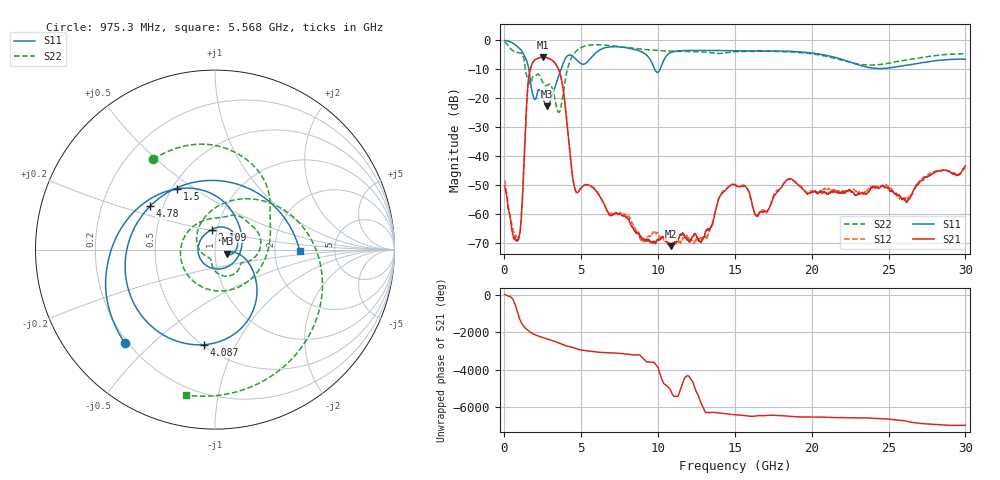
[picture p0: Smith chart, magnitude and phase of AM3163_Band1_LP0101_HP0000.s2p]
!Agilent Technologies,E8364B,MY43040894,A.07.50.67
!Agilent E8364B: A.07.50.67
!Date: Thursday, August 20, 2020 11:26:09
!Correction: S11(Full 2 Port(1,2))
!S21(Full 2 Port(1,2))
!S12(Full 2 Port(1,2))
!S22(Full 2 Port(1,2))
!S2P File: Measurements: S11, S21, S12, S22:
# Hz S  dB  R 50
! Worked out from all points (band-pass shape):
!   3201 points, 10 MHz to 30 GHz, reference 50 ohm
!   highest |S21| = -5.82 dB at 2.512 GHz (marker M1); lowest = -71.3 dB at 10.86 GHz (marker M2)
!   |S21| within 3 dB of the highest: 1.752 GHz to 3.411 GHz (1.659 GHz wide, 64.3 % of centre)
!   lowest |S11| = -22.8 dB at 2.775 GHz (marker M3), VSWR 1.16, Z = 57.4 - j2.53 ohm
!   |S11| at or under -10 dB: 1.588 GHz to 3.688 GHz (2.099 GHz wide, 79.6 % of centre); 9.776 GHz to 10.13 GHz (355.8 MHz wide, 3.57 % of centre)
!   |S22| runs from -24.9 to -0.6 dB; largest |S21 - S12| = 0.0029
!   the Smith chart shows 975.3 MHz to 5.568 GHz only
!   S11 on the Smith chart (normalised r, x): 975.3 MHz: 0.19, -0.41; 1.5 GHz: 0.53, +0.43; 2.109 GHz: 0.94, +0.21; 4.087 GHz: 0.51, -0.75; 4.78 GHz: 0.42, +0.25; 5.568 GHz: 2.79, -0.06
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1e7  -0.07 -8.8  -50.49 19.2  -48.45 10.2  -0.56 -25.3
5.067094e8  -0.89 -67.4  -66.45 -177.0  -64.48 -128.6  -3.46 -148.5
9.753031e8  -2.81 -134.1  -67.27 175.2  -68.07 -151.9  -4.30 124.3
1.500128e9  -7.99 121.9  -17.45 -73.9  -17.42 -74.1  -13.02 -102.6
2.1093e9  -18.93 99.1  -6.41 -10.6  -6.41 -10.7  -11.83 23.5
2.512291e9  -20.08 -13.8  -5.82 -126.5  -5.82 -126.6  -14.88 -22.8
2.774703e9  -22.80 -17.6  -6.04 164.6  -6.05 164.5  -15.57 -32.6
3.318272e9  -15.54 -15.3  -8.08 19.6  -8.10 19.6  -21.40 -101.3
4.086766e9  -5.46 -96.8  -29.48 139.1  -29.46 139.4  -10.33 66.5
4.780284e9  -7.23 146.1  -52.66 -27.1  -52.62 -26.9  -3.25 -35.4
5.014581e9  -8.19 101.4  -51.03 -70.2  -50.84 -69.8  -2.47 -57.9
5.567522e9  -6.51 -0.9  -50.29 -133.7  -50.37 -134.2  -1.66 -101.3
6.392247e9  -2.87 -95.7  -55.67 154.4  -55.85 152.3  -1.62 -150.9
7.451269e9  -2.29 -169.4  -60.24 114.6  -60.14 112.7  -2.18 159.1
1.000979e10  -11.00 96.8  -68.99 41.3  -67.02 95.8  -3.53 59.7
1.086263e10  -4.20 75.3  -71.26 -143.7  -70.41 -71.4  -3.76 29.4
1.256831e10  -3.52 1.3  -68.29 101.0  -68.89 141.7  -3.98 -27.3
1.5005e10  -3.63 -72.2  -49.97 66.8  -50.23 67.4  -3.95 -90.6
2.000958e10  -4.42 163.2  -52.54 -57.2  -52.17 -54.7  -4.69 136.3
2.275554e10  -8.02 60.0  -53.22 -102.4  -51.63 -99.0  -7.98 21.1
2.500479e10  -9.61 -62.1  -51.35 -163.2  -50.65 -170.8  -7.97 -92.5
3e10  -6.61 104.4  -43.45 -135.9  -44.06 -133.9  -4.63 102.0
